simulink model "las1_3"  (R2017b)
settings: Solver=ode45  StartTime=0.0  StopTime=300  MaxStep=1  RelTol=1e-3  AbsTol=1e-3
undefined symbols (not defined in the file): A, B, C, D, y0

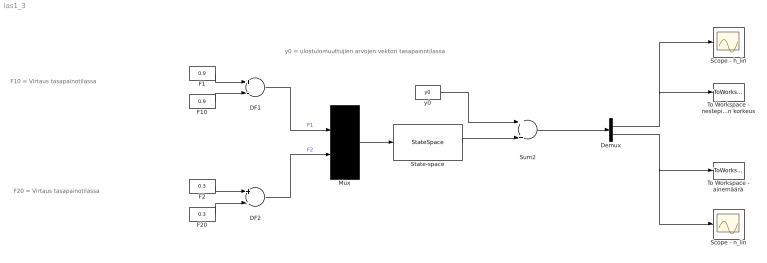
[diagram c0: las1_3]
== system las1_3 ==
  note: F10 = Virtaus tasapainotilassa
  note: F20 = Virtaus tasapainotilassa
  note: y0 = ulostulomuuttujien arvojen vektori tasapainotilassa
  DF1 : Sum  Inputs=+-
  DF2 : Sum  Inputs=+-
  Demux : Demux  Outputs=2
  F1 : Constant  Value=0.9
  F10 : Constant  Value=0.9
  F2 : Constant  Value=0.3
  F20 : Constant  Value=0.3
  Mux : Mux  Inputs=2
  Scope - h_lin : Scope
  Scope - n_lin : Scope
  State-space : StateSpace  A=A  B=B  C=C  D=D  InitialCondition=[0 0]
  Sum2 : Sum
  To Workspace - ainemäärä : ToWorkspace  VariableName=n_lin
  To Workspace - nestepinnan korkeus : ToWorkspace  VariableName=h_lin
  y0 : Constant  Value=y0
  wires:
  State-space/1 -> Sum2/2
  y0/1 -> Sum2/1
  F20/1 -> DF2/2
  F2/1 -> DF2/1
  F10/1 -> DF1/2
  F1/1 -> DF1/1
  DF2/1 -> Mux/2  "F2"
  DF1/1 -> Mux/1  "F1"
  Mux/1 -> State-space/1
  Sum2/1 -> Demux/1
  Demux/1 -> To Workspace - nestepinnan korkeus/1, Scope - h_lin/1
  Demux/2 -> To Workspace - ainemäärä/1, Scope - n_lin/1
